FUNCTION_BLOCK FB 10
TITLE =
VERSION : 0.1


VAR_INPUT
  START : BOOL ;
  S1 : BOOL ;
  S2 : BOOL ;
  S3 : BOOL ;
  S4 : BOOL ;
  S5 : BOOL ;
  RESET : BOOL ;
  Zeit_1 : TIMER ;
  Zeitw_1 : S5TIME  := S5T#10S;
  Zeit_2 : TIMER ;
  Zeitw_2 : S5TIME  := S5T#5S;
END_VAR
VAR_OUTPUT
  Y1 : BOOL ;
  Y2 : BOOL ;
  Y3 : BOOL ;
  Y4 : BOOL ;
  H : BOOL ;
  M : BOOL ;
END_VAR
VAR
  SRO_1 : BOOL  := TRUE;
  SRO_2 : BOOL ;
  SRO_3 : BOOL ;
  SRO_4 : BOOL ;
  SRO_5 : BOOL ;
  SRO_6 : BOOL ;
END_VAR
BEGIN
NETWORK
TITLE =
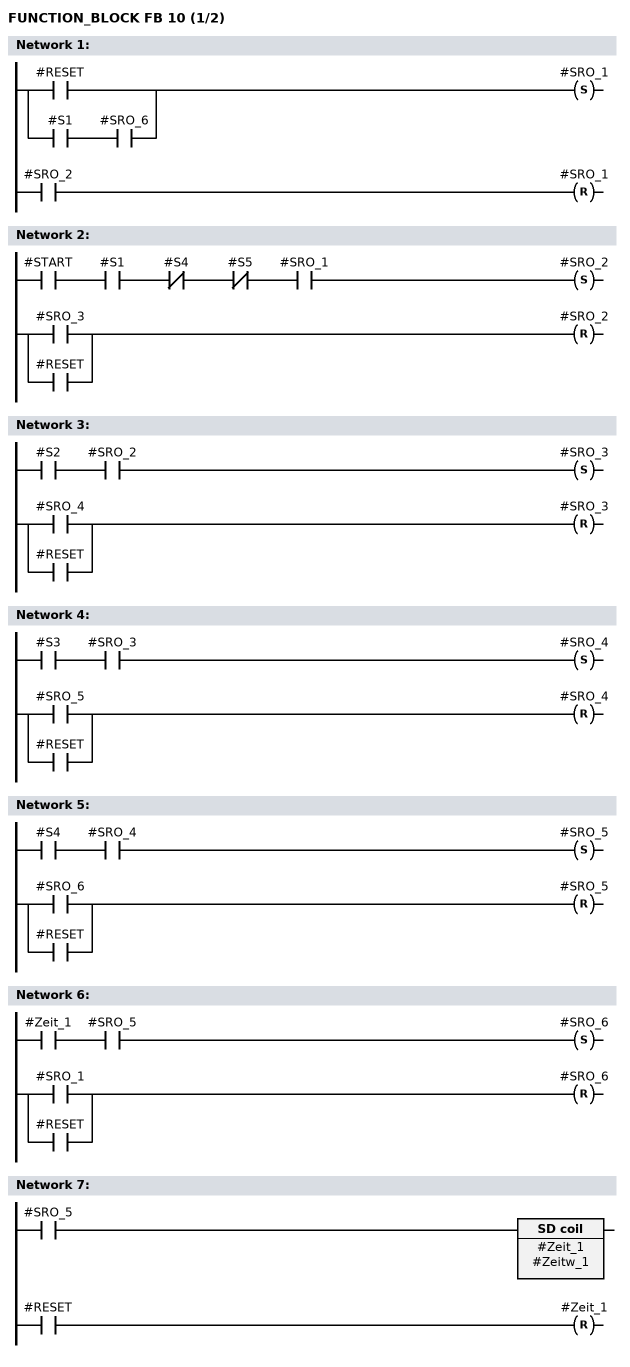
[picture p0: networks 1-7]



      U(    ;
      O     #RESET;
      O     ;
      U     #S1;
      U     #SRO_6;
      )     ;
      S     #SRO_1;
      U     #SRO_2;
      R     #SRO_1;
      NOP   0;
NETWORK
TITLE =

      U     #START;
      U     #S1;
      UN    #S4;
      UN    #S5;
      U     #SRO_1;
      S     #SRO_2;
      U(    ;
      O     #SRO_3;
      O     #RESET;
      )     ;
      R     #SRO_2;
      NOP   0;
NETWORK
TITLE =

      U     #S2;
      U     #SRO_2;
      S     #SRO_3;
      U(    ;
      O     #SRO_4;
      O     #RESET;
      )     ;
      R     #SRO_3;
      NOP   0;
NETWORK
TITLE =

      U     #S3;
      U     #SRO_3;
      S     #SRO_4;
      U(    ;
      O     #SRO_5;
      O     #RESET;
      )     ;
      R     #SRO_4;
      NOP   0;
NETWORK
TITLE =

      U     #S4;
      U     #SRO_4;
      S     #SRO_5;
      U(    ;
      O     #SRO_6;
      O     #RESET;
      )     ;
      R     #SRO_5;
      NOP   0;
NETWORK
TITLE =

      U     #Zeit_1;
      U     #SRO_5;
      S     #SRO_6;
      U(    ;
      O     #SRO_1;
      O     #RESET;
      )     ;
      R     #SRO_6;
      NOP   0;
NETWORK
TITLE =

      U     #SRO_5;
      L     #Zeitw_1;
      SE    #Zeit_1;
      U     #RESET;
      R     #Zeit_1;
      NOP   0;
      NOP   0;
      NOP   0;
NETWORK
TITLE =
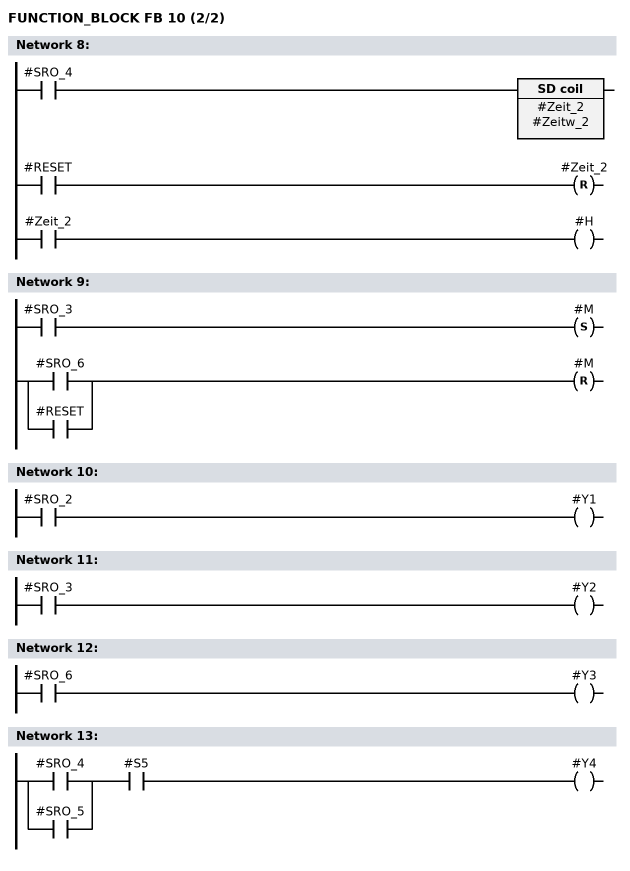
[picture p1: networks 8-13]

      U     #SRO_4;
      L     #Zeitw_2;
      SE    #Zeit_2;
      U     #RESET;
      R     #Zeit_2;
      NOP   0;
      NOP   0;
      U     #Zeit_2;
      =     #H;
NETWORK
TITLE =

      U     #SRO_3;
      S     #M;
      U(    ;
      O     #SRO_6;
      O     #RESET;
      )     ;
      R     #M;
      NOP   0;
NETWORK
TITLE =

      U     #SRO_2;
      =     #Y1;
NETWORK
TITLE =

      U     #SRO_3;
      =     #Y2;
NETWORK
TITLE =

      U     #SRO_6;
      =     #Y3;
NETWORK
TITLE =

      U(    ;
      O     #SRO_4;
      O     #SRO_5;
      )     ;
      U     #S5;
      =     #Y4;
END_FUNCTION_BLOCK

